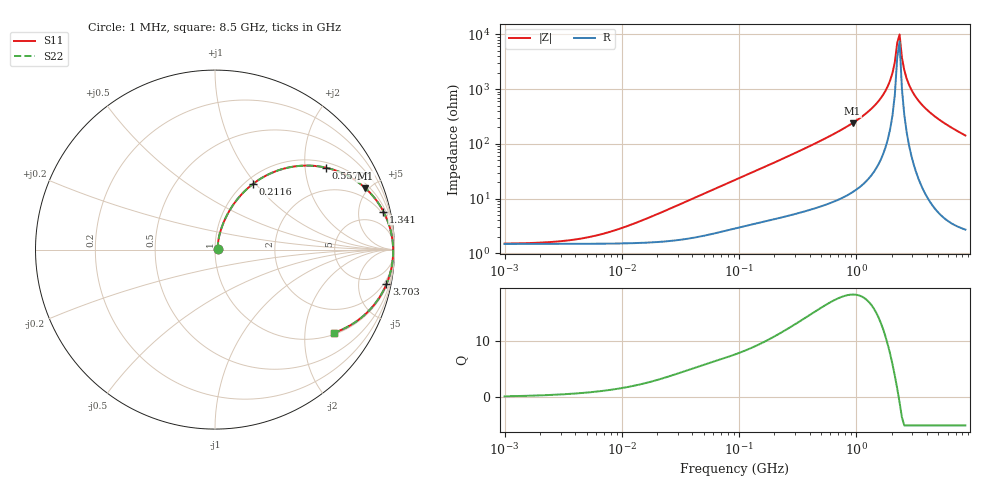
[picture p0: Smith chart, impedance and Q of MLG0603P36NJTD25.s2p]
! S-Parameter Data Generated by TDK Corporation
! Copyright(C) 2025 TDK Corporation.
! All Rights Reserved.
! TDK P/N: MLG0603P36NJTD25 (SMD / SMT Inductor (Coil))
! Property: L=36nH at 300MHz
! Size(LxWxT): 0.6x0.3x0.3mm
! Model Type: s2p (Touchstone File Format Version 1.0)
! Frequency: DC=Yes Start=1MHz Stop=8500MHz 198points Log-sweep
! Model Generated on Feb. 6, 2025
! Terms and conditions regarding TDK Simulation Models:
! 1)This simulation model is being provided solely for informational
!  purposes. Please refer to the specifications of the products in
!  terms of detailed characteristics of such products.
! 2)In no event shall TDK Corporation of any of its subsidiaries be
!  liable for any loss or damage arising, directly or indirectly,
!  from any information contained in this simulation model, including,
!  but not limited to loss or damages arising from any inaccuracies,
!  omissions or errors in connection with such information.
! 3)Any and all copyrights on this simulation model are owned by
!  TDK Corporation.  Duplication or redistribution of this simulation
!  model without prior written permission from TDK Corporation
!  is prohibited.
! 4)This simulation model is subject to any modification or change
!  without any prior notice.
! 5)Neither TDK Corporation nor any of its subsidiaries shall make any
!  warranty, express or implied, including but not limited to the
!  correctness, implied warranties of merchantability and fitness for
!  a particular purpose with respect to this simulation models.
! 6)The use of this simulation model shall be deemed to have consented
!  to the terms and conditions hereof.
! Port Assignments:
!  1 ---@@@--- 2
! Applicable Conditions:
!  Temperature = 25 degC
!  DC Bias Current = 0 A
!  Small Signal Operation
# Hz S MA R 50
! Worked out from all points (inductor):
!   197 points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, 1 MHz to 8.5 GHz, reference 50 ohm
!   read as one part in series: L = 39.3 nH near 20.1 MHz
!   highest Q = 18.2 at 927.1 MHz (marker M1), where L = 41 nH
!   self-resonance near 2.229 GHz
!   S11 on the Smith chart (normalised r, x): 1 MHz: 1.03, +0.00; 211.6 MHz: 1.09, +0.96; 557.9 MHz: 1.16, +2.59; 1.341 GHz: 1.53, +8.72; 3.703 GHz: 1.29, -9.84; 8.5 GHz: 1.05, -2.84
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1000000  0.01489 9.3  0.9853 -0.1  0.9853 -0.1  0.01489 9.3
4587603  0.01854 36.7  0.9852 -0.6  0.9852 -0.6  0.01854 36.7
9168677  0.02694 55.1  0.9848 -1.3  0.9848 -1.3  0.02694 55.1
2.10461e7  0.05356 69.7  0.9827 -2.9  0.9827 -2.9  0.05356 69.7
9.219544e7  0.208 70.6  0.9514 -11.9  0.9514 -11.9  0.208 70.6
2.116287e8  0.4202 60.1  0.8704 -24.7  0.8704 -24.7  0.4202 60.1
4.229561e8  0.6723 44.0  0.6967 -42.1  0.6967 -42.1  0.6723 44.0
5.57935e8  0.7696 36.3  0.5936 -50.2  0.5936 -50.2  0.7696 36.3
9.270694e8  0.9052 22.2  0.3782 -64.7  0.3782 -64.7  0.9052 22.2
1.34121e9  0.9621 12.7  0.2201 -73.8  0.2201 -73.8  0.9621 12.7
1.689417e9  0.982 7.1  0.1247 -78.1  0.1247 -78.1  0.982 7.1
1.940355e9  0.9888 3.9  0.06858 -78.7  0.06858 -78.7  0.9888 3.9
2.128028e9  0.9914 1.8  0.03171 -73.5  0.03171 -73.5  0.9914 1.8
2.228565e9  0.9922 0.7  0.01428 -56.5  0.01428 -56.5  0.9922 0.7
2.333852e9  0.9925 -0.4  0.009987 41.5  0.009987 41.5  0.9925 -0.4
2.444114e9  0.9925 -1.5  0.02637 72.8  0.02637 72.8  0.9925 -1.5
2.559585e9  0.9921 -2.5  0.04468 78.6  0.04468 78.6  0.9921 -2.5
2.680511e9  0.9913 -3.6  0.06332 80.3  0.06332 80.3  0.9913 -3.6
3.07866e9  0.9866 -6.9  0.1202 80.2  0.1202 80.2  0.9866 -6.9
3.703002e9  0.9743 -11.4  0.198 76.9  0.198 76.9  0.9743 -11.4
5.357206e9  0.9257 -21.2  0.3613 67.8  0.3613 67.8  0.9257 -21.2
8.5e9  0.8104 -34.8  0.5705 54.1  0.5705 54.1  0.8104 -34.8
